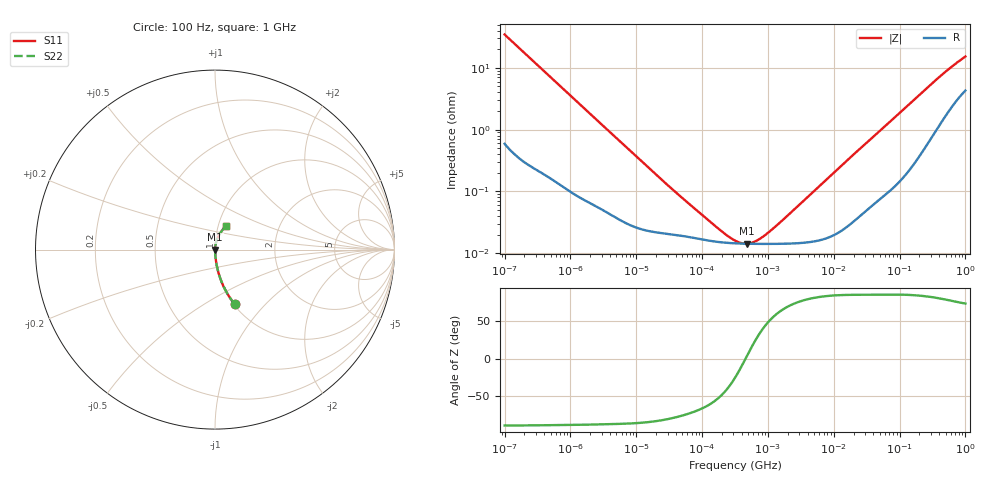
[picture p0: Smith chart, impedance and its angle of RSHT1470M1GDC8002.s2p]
! RSHT1470M1GDC8002  S-PARAMETER MODEL  (General Type)
! Model Generated by ELNA Corporation (http://www.ty-top.com)
! Version 1.0
! ELNA Control No.201026
! Copyright (c) 2020 ELNA CO.,LTD. All Rights Reserved.
! Products Name : CONDUCTIVE POLYMER HYBRID ALUMINUM ELECTROLYTIC CAPACITORS
! Characteristics :
!  Capacitance  :  47uF  ,  Rated voltage  :  35V
!  Operating Temp. Range  :  -55 to +105 degC  ,  Endurance  :  5000hr at 105 degC
!  Dimension D  :  6.3mm  ,  Dimension L  :  5.8mm
! Frequency Range : 100Hz - 1GHz
! External Node Assignments :
!  1  o---| |---o  2
# MHz S RI R 50
!Freq[MHz].  S11 Real  S11 Imag  S21 Real  S21 Imag  S12 Real  S12 Imag  S22 Real  S22 Imag
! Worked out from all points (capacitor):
!   401 points, 100 Hz to 1 GHz, reference 50 ohm
!   read as one part in series: C = 46 uF near 108 Hz
!   lowest |Z| = 14.3 mohm at 473.2 kHz (marker M1)
!   series resonance near 457 kHz, so ESL is about 2.6 nH
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0.0001  0.1111 -0.3058  0.8889 0.3058  0.8889 0.3058  0.1111 -0.3058
0.000113  0.0899 -0.2778  0.9101 0.2778  0.9101 0.2778  0.0899 -0.2778
0.000169  0.0434 -0.1957  0.9566 0.1957  0.9566 0.1957  0.0434 -0.1957
0.000335  0.0127 -0.1025  0.9873 0.1025  0.9873 0.1025  0.0127 -0.1025
0.000638  0.00436 -0.0547  0.9956 0.0547  0.9956 0.0547  0.00436 -0.0547
0.001488  0.00133 -0.0239  0.9987 0.0239  0.9987 0.0239  0.00133 -0.0239
0.022131  0.000217 -0.00168  0.9998 0.00168  0.9998 0.00168  0.000217 -0.00168
0.049545  0.000192 -0.000765  0.9998 0.000765  0.9998 0.000765  0.000192 -0.000765
0.165959  0.000153 -0.000215  0.9998 0.000215  0.9998 0.000215  0.000153 -0.000215
0.238506  0.000147 -0.000127  0.9999 0.000127  0.9999 0.000127  0.000147 -0.000127
0.316228  0.000145 -6.89e-05  0.9999 6.89e-05  0.9999 6.89e-05  0.000145 -6.89e-05
0.386812  0.000143 -3.07e-05  0.9999 3.07e-05  0.9999 3.07e-05  0.000143 -3.07e-05
0.473151  0.000142 6.41e-06  0.9999 -6.41e-06  0.9999 -6.41e-06  0.000142 6.41e-06
0.653131  0.000142 6.72e-05  0.9999 -6.72e-05  0.9999 -6.72e-05  0.000142 6.72e-05
0.938642  0.000141 0.000144  0.9999 -0.000144  0.9999 -0.000144  0.000141 0.000144
1.584893  0.000142 0.000293  0.9999 -0.000293  0.9999 -0.000293  0.000142 0.000293
4.704354  0.000154 0.000939  0.9998 -0.000939  0.9998 -0.000939  0.000154 0.000939
69.9842  0.00117 0.0131  0.9988 -0.0131  0.9988 -0.0131  0.00117 0.0131
176.8072  0.00408 0.0321  0.9959 -0.0321  0.9959 -0.0321  0.00408 0.0321
395.8221  0.0159 0.0673  0.9841 -0.0673  0.9841 -0.0673  0.0159 0.0673
695.825  0.0379 0.1044  0.9621 -0.1044  0.9621 -0.1044  0.0379 0.1044
1000  0.0595 0.1317  0.9405 -0.1317  0.9405 -0.1317  0.0595 0.1317
